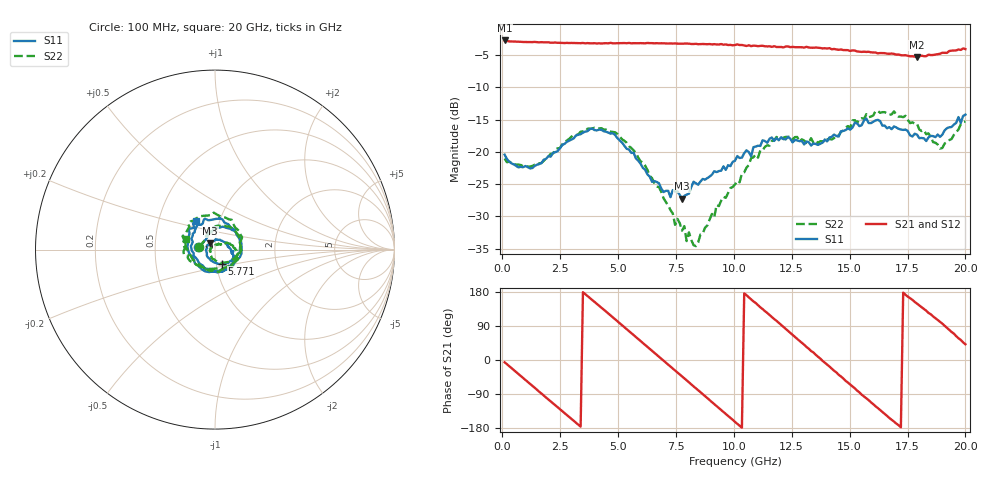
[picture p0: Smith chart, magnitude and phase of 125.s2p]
!Agilent Technologies,N5230C,MY49001569,A.09.33.09
!Agilent N5230C: A.09.33.09
!Date: Tuesday, July 28, 2015 11:14:15
!Correction: S11(Full 2 Port(1,2))
!S21(Full 2 Port(1,2))
!S12(Full 2 Port(1,2))
!S22(Full 2 Port(1,2))
!S2P File: Measurements: S11, S21, S12, S22:
# Hz S  dB  R 50
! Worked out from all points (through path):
!   201 points, 100 MHz to 20 GHz, reference 50 ohm
!   highest |S21| = -2.73 dB at 100 MHz (marker M1); lowest = -5.3 dB at 17.91 GHz (marker M2)
!   group delay of S21, straight-line fit = 145 ps
!   lowest |S11| = -27.2 dB at 7.761 GHz (marker M3), VSWR 1.09, Z = 47.3 + j3.29 ohm
!   |S11| at or under -10 dB: start of sweep to end of sweep
!   |S22| runs from -34.6 to -13.6 dB; largest |S21 - S12| = 0.024
!   S11 on the Smith chart (normalised r, x): 100 MHz: 0.83, +0.03; 5.771 GHz: 1.07, -0.17; 20 GHz: 0.77, +0.26
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1e8  -20.43 170.7  -2.73 -6.0  -2.79 -5.5  -21.02 169.2
9.955e8  -22.20 140.2  -2.97 -52.5  -2.96 -52.7  -22.20 144.8
1.7915e9  -21.21 119.2  -3.02 -93.8  -3.05 -93.7  -21.39 125.7
2.687e9  -18.76 91.6  -3.13 -140.0  -3.06 -140.3  -18.49 99.6
3.483e9  -17.03 57.1  -3.12 178.9  -3.18 178.7  -16.82 67.7
4.677e9  -17.18 0.4  -3.10 117.6  -3.18 117.4  -16.86 11.7
5.7715e9  -21.02 -63.3  -3.16 60.8  -3.17 60.5  -20.16 -45.3
6.7665e9  -24.87 -142.3  -3.18 8.7  -3.15 8.7  -25.46 -105.0
7.7615e9  -27.25 127.0  -3.24 -43.2  -3.24 -43.6  -32.22 174.0
8.3585e9  -24.85 81.0  -3.25 -74.8  -3.32 -74.7  -34.62 118.7
8.856e9  -24.07 50.6  -3.32 -100.6  -3.33 -101.0  -31.40 74.5
1.005e10  -21.38 2.9  -3.45 -163.3  -3.48 -163.4  -25.05 36.7
1.1045e10  -19.05 -19.0  -3.62 144.9  -3.51 144.9  -20.90 17.7
1.19405e10  -18.21 -50.8  -3.74 98.1  -3.65 97.3  -17.92 -19.6
1.3433e10  -18.71 -136.1  -3.86 20.1  -3.94 18.4  -18.56 -88.1
1.41295e10  -17.75 -176.9  -3.92 -17.1  -4.04 -17.8  -18.03 -125.9
1.51245e10  -16.23 137.1  -4.27 -69.8  -4.26 -70.7  -15.13 -171.8
1.5821e10  -15.53 102.6  -4.49 -105.8  -4.56 -106.7  -14.63 150.9
1.67165e10  -16.17 45.0  -4.79 -153.1  -4.88 -152.7  -14.23 102.8
1.79105e10  -17.33 -51.9  -5.29 148.8  -5.21 147.7  -15.63 24.0
1.9005e10  -17.32 -163.0  -4.64 95.8  -4.78 95.0  -19.40 -92.6
2e10  -14.22 123.8  -4.07 41.5  -4.04 41.4  -15.30 160.0
